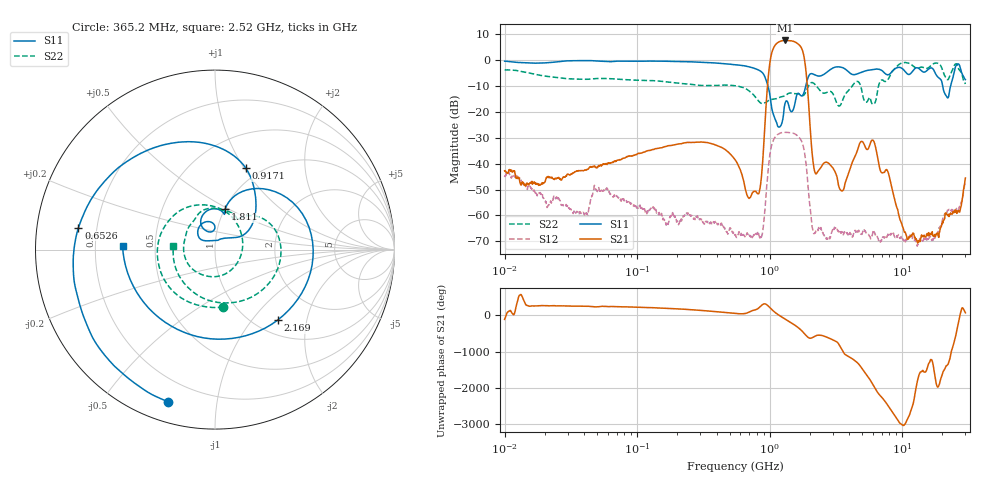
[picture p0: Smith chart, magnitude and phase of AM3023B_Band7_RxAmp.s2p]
# Hz S DB R 50.0
!freq dBS11 angS11 dBS21 angS21 dBS12 angS12 dBS22 angS22
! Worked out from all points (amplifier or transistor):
!   1601 points, 10 MHz to 30 GHz, reference 50 ohm
!   highest |S21| = 7.6 dB at 1.308 GHz (marker M1)
!   |S21| within 3 dB of that: 1.068 GHz to 1.742 GHz (674 MHz wide, 48 % of centre)
!   unconditionally stable (mu >= 1): start of sweep to end of sweep
!   at 37.85 MHz: K = 2251.38, MAG = -28.5 dB, |S12| = -58.7 dB
!   at 547.7 MHz: K = 30827.31, MAG = -33.3 dB, |S12| = -67.6 dB
!   at 30 GHz: K = 15214.73, MAG = -44.2 dB, |S12| = -46.9 dB
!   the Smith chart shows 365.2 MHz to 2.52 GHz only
!   S11 on the Smith chart (normalised r, x): 365.2 MHz: 0.09, -0.73; 652.6 MHz: 0.13, +0.08; 917.1 MHz: 0.86, +1.02; 1.811 GHz: 1.01, +0.48; 2.169 GHz: 1.25, -1.36; 2.52 GHz: 0.32, +0.02
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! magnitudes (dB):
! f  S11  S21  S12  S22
! 10 MHz  -0.4  -42.8  -45.2  -3.8
! 38.04 MHz  -0.2  -42.6  -58.7  -7.4
! 49.35 MHz  -0.3  -41.7  -50.2  -7.1
! 144.7 MHz  -0.4  -34.1  -59.7  -8.1
! 365.2 MHz  -1.0  -32.3  -63.2  -9.8
! 547.7 MHz  -1.8  -38.4  -67.6  -9.9
! 652.6 MHz  -2.3  -49.3  -68.2  -10.9
! 829.7 MHz  -3.9  -51.4  -67.3  -16.0
! 917.1 MHz  -6.3  -26.7  -58.7  -16.5
! 1.034 GHz  -18.3  2.5  -32.9  -15.2
! 1.308 GHz  -16.6  7.6  -27.9  -13.8
! 1.811 GHz  -12.7  1.7  -34.2  -13.5
! 2.084 GHz  -5.2  -35.0  -63.9  -8.7
! 2.169 GHz  -5.6  -42.2  -67.1  -9.1
! 2.52 GHz  -5.8  -40.2  -66.7  -12.7
! 3.524 GHz  -2.9  -50.5  -66.4  -16.0
! 5.989 GHz  -3.7  -30.9  -66.9  -17.1
! 7.926 GHz  -5.6  -44.2  -67.6  -7.0
! 13.14 GHz  -3.0  -70.2  -71.3  -3.1
! 21.67 GHz  -14.1  -59.5  -59.1  -7.3
! 25.95 GHz  -1.6  -58.9  -58.4  -1.6
! 30 GHz  -7.5  -45.6  -46.9  -9.2
